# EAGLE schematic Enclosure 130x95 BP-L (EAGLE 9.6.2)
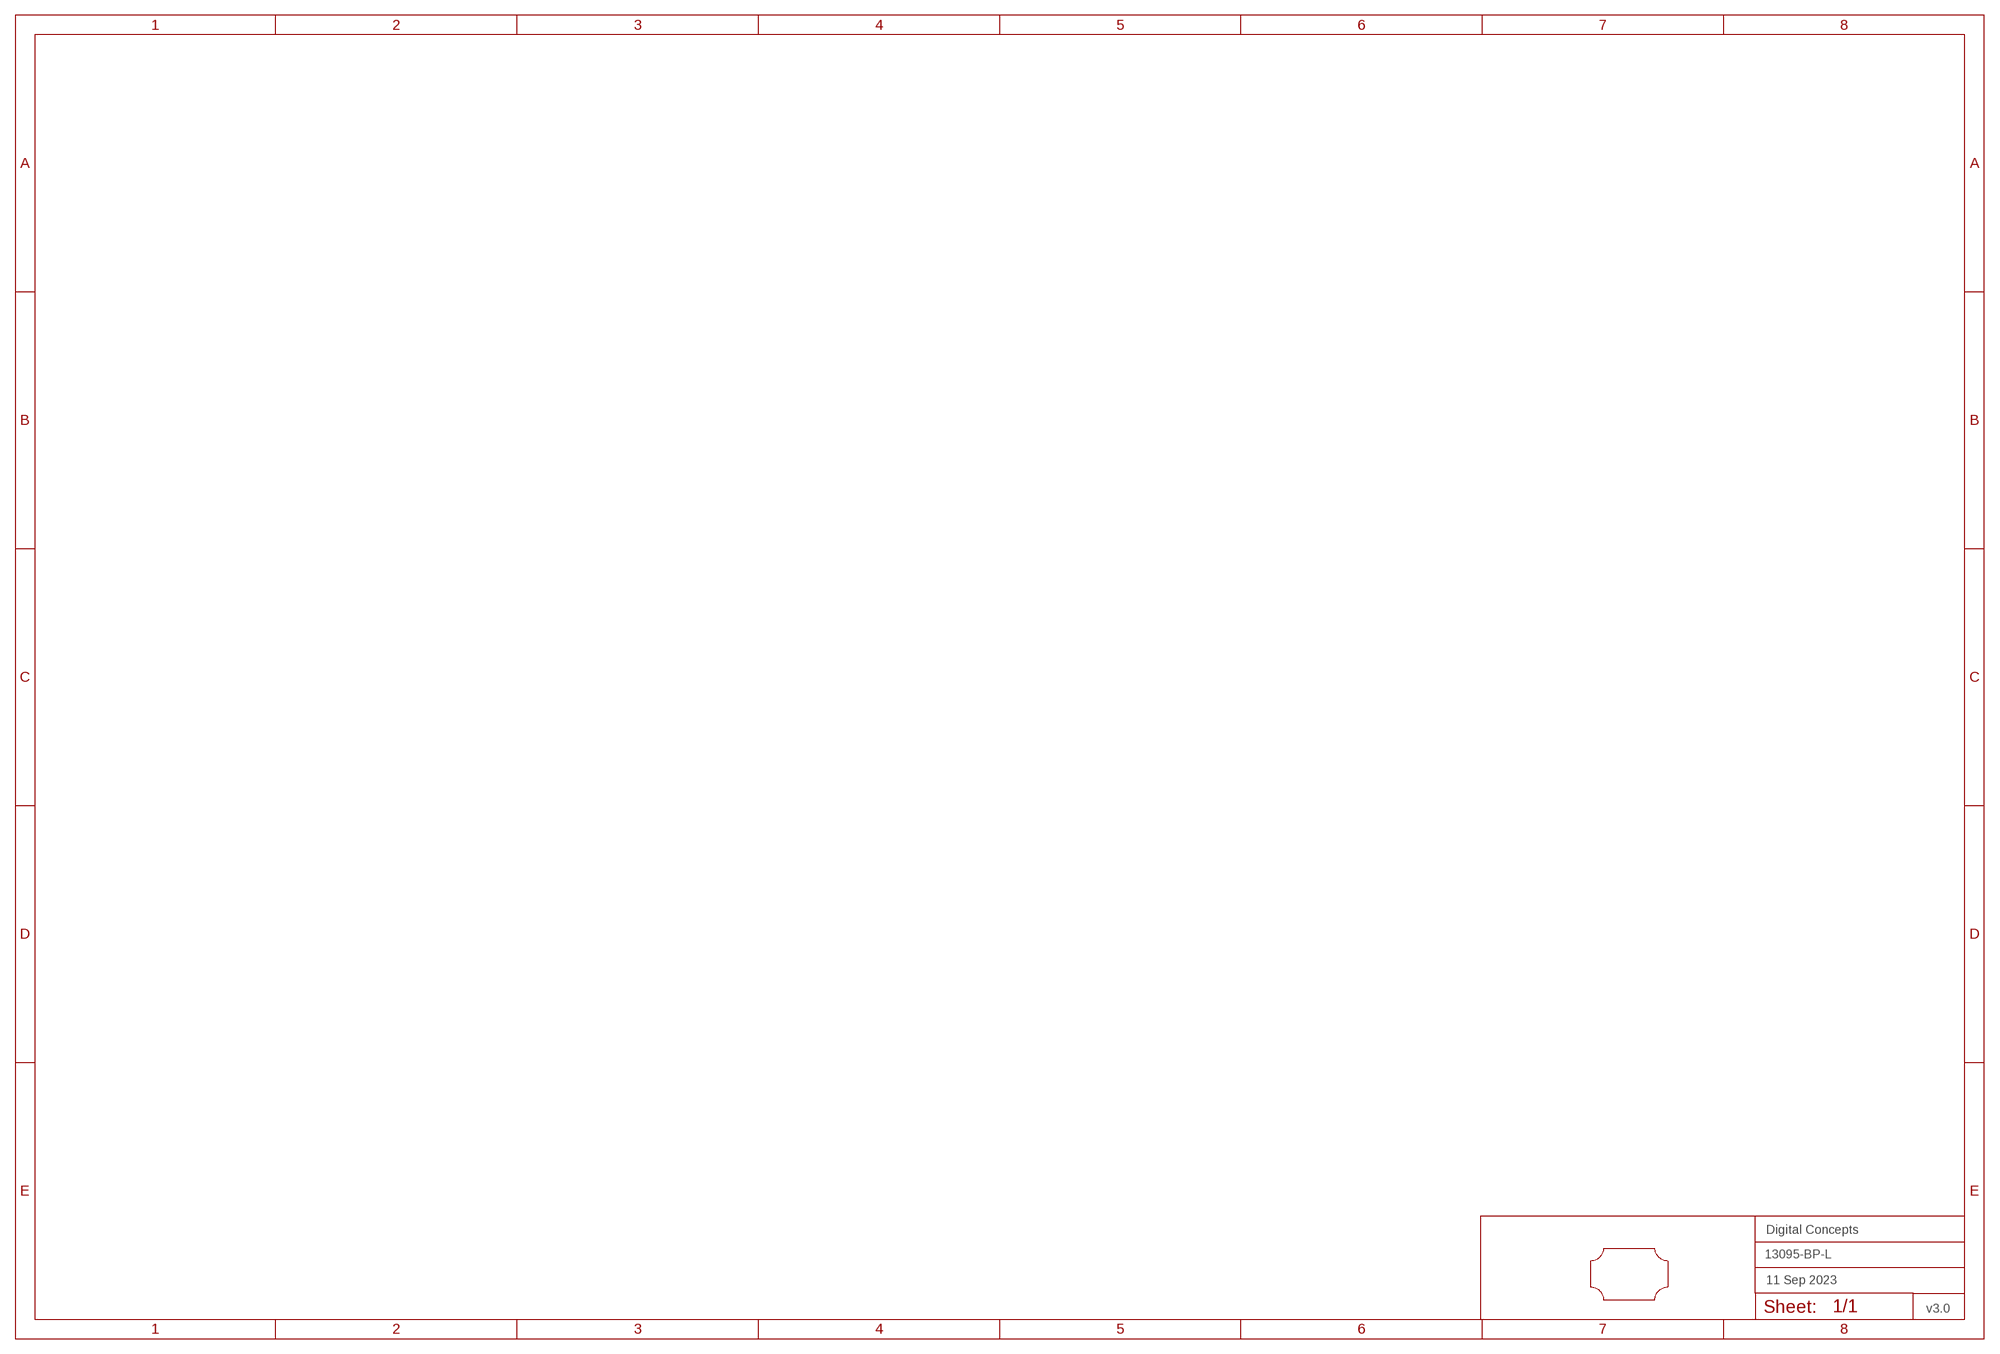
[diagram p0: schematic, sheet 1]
FRAME2 (A3L-LOC): DATE: 11 Sep 2023; OWNER: Digital Concepts; TITLE: 13095-BP-L; VERSION: v3.0

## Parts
U$1  PCB-OUTLINE-130X95-MAX-LC-H3  [PROTO-130X95-OUTLINE-MAX-LC-H3]

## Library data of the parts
U$1 = digitalconcepts:PCB-OUTLINE-130X95-MAX-LC-H3: PCB Eagle Max-Left-Cropped outline for 130 x 95 enclosure (Horizontal format)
